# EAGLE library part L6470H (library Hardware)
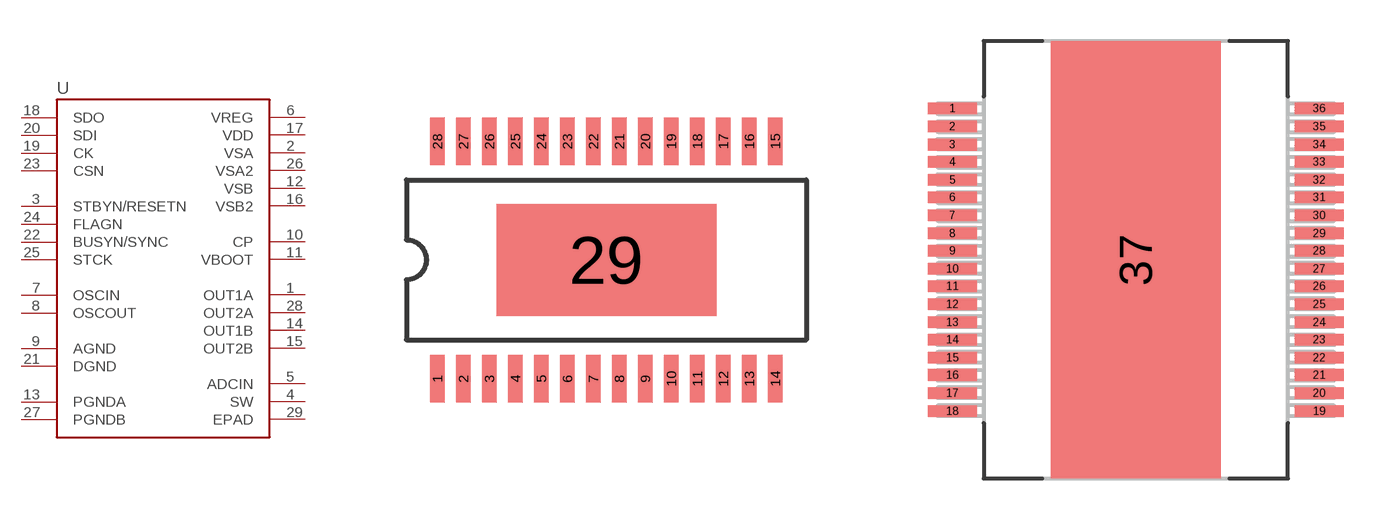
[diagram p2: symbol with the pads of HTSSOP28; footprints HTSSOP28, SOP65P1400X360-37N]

Designator prefix -

## L6470HHTSSOP28  [HTSSOP28]
1  OUT1A
2  VSA
3  STBYN/RESETN
4  SW
5  ADCIN
6  VREG
7  OSCIN
8  OSCOUT
9  AGND
10  CP
11  VBOOT
12  VSB
13  PGNDA
14  OUT1B
15  OUT2B
16  VSB2
17  VDD
18  SDO
19  CK
20  SDI
21  DGND
22  BUSYN/SYNC
23  CSN
24  FLAGN
25  STCK
26  VSA2
27  PGNDB
28  OUT2A
29  EPAD

## L6470HPOWERSO36  [SOP65P1400X360-37N]
1  PGNDA
2  OUT1A
3  OUT1A
4  VSA
5  VSA
6  STBYN/RESETN
7  SW
8  ADCIN
9  VREG
10  OSCIN
11  OSCOUT
12  AGND
13  CP
14  VBOOT
15  VSB
16  VSB
17  OUT1B
18  OUT1B
19  PGNDB
20  OUT2B
21  OUT2B
22  VSB2
23  VSB2
24  VDD
25  SDO
26  CK
27  SDI
28  DGND
29  BUSYN/SYNC
30  CSN
31  FLAGN
32  STCK
33  VSA2
34  VSA2
35  OUT2A
36  OUT2A
37  EPAD

## Footprint HTSSOP28 (pad centres in mm)
smd 0.36 x 1.19: 1 -4.225,-2.97; 2 -3.575,-2.97; 3 -2.925,-2.97; 4 -2.275,-2.97; 5 -1.625,-2.97; 6 -0.975,-2.97; 7 -0.325,-2.97; 8 0.325,-2.97; 9 0.975,-2.97; 10 1.625,-2.97; 11 2.275,-2.97; 12 2.925,-2.97; 13 3.575,-2.97; 14 4.225,-2.97; 15 4.225,2.97; 16 3.575,2.97; 17 2.925,2.97; 18 2.275,2.97; 19 1.625,2.97; 20 0.975,2.97; 21 0.325,2.97; 22 -0.325,2.97; 23 -0.975,2.97; 24 -1.625,2.97; 25 -2.275,2.97; 26 -2.925,2.97; 27 -3.575,2.97; 28 -4.225,2.97
smd 5.5 x 2.8: 29 0,0

## Footprint SOP65P1400X360-37N (pad centres in mm)
smd 1.803 x 0.432: 1 -6.706,5.537; 2 -6.706,4.877; 3 -6.706,4.216; 4 -6.706,3.581; 5 -6.706,2.921; 6 -6.706,2.286; 7 -6.706,1.626; 8 -6.706,0.965; 9 -6.706,0.33; 10 -6.706,-0.33; 11 -6.706,-0.965; 12 -6.706,-1.626; 13 -6.706,-2.286; 14 -6.706,-2.921; 15 -6.706,-3.581; 16 -6.706,-4.216; 17 -6.706,-4.877; 18 -6.706,-5.537; 19 6.706,-5.537; 20 6.706,-4.877; 21 6.706,-4.216; 22 6.706,-3.581; 23 6.706,-2.921; 24 6.706,-2.286; 25 6.706,-1.626; 26 6.706,-0.965; 27 6.706,-0.33; 28 6.706,0.33; 29 6.706,0.965; 30 6.706,1.626; 31 6.706,2.286; 32 6.706,2.921; 33 6.706,3.581; 34 6.706,4.216; 35 6.706,4.877; 36 6.706,5.537
smd 6.198 x 16.002: 37 0,0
